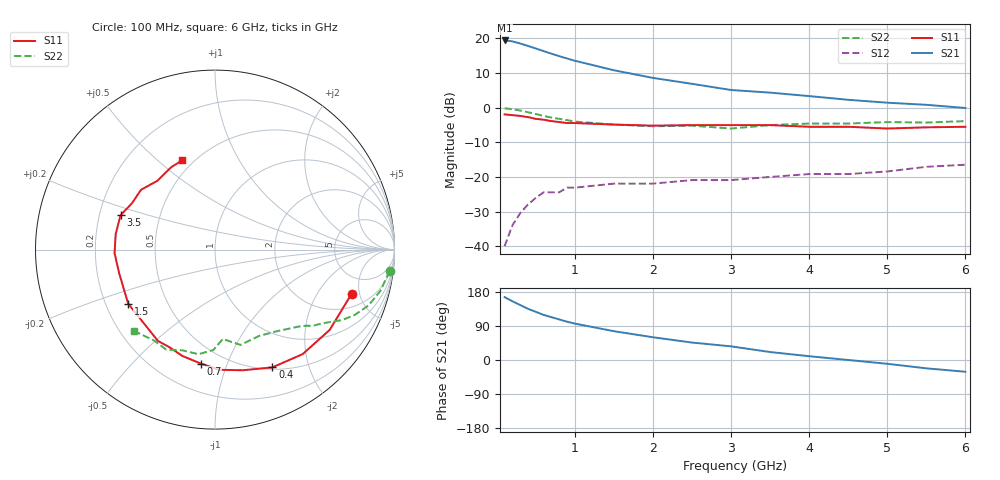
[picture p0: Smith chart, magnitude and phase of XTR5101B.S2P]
! HXTR-5101  (2N6701) Common Emitter
! Vce=15V  Ic=15mA
# ghz s ma r 50
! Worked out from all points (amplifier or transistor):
!   20 points, 100 MHz to 6 GHz, reference 50 ohm
!   highest |S21| = 19.4 dB at 100 MHz (marker M1)
!   |S21| within 3 dB of that: start of sweep to 589.7 MHz
!   unconditionally stable (mu >= 1): 1.896 GHz to end of sweep
!   at 400 MHz: K = 0.25, MSG = 22.9 dB, |S12| = -28.0 dB
!   at 1.5 GHz: K = 0.79, MSG = 16.4 dB, |S12| = -21.9 dB
!   at 6 GHz: K = 1.17, MAG = 5.7 dB, |S12| = -16.5 dB
!   S11 on the Smith chart (normalised r, x): 100 MHz: 3.04, -4.18; 400 MHz: 0.52, -1.47; 700 MHz: 0.38, -0.81; 1.5 GHz: 0.29, -0.26; 3.5 GHz: 0.29, +0.16; 6 GHz: 0.44, +0.61
0.1  0.8 -18.0  9.35 166.0  0.01 78.0  0.98 -7.0
0.2  0.78 -35.0  9.07 155.0  0.02 69.0  0.95 -14.0
0.3  0.76 -50.0  8.44 145.0  0.03 61.0  0.91 -20.0
0.4  0.73 -64.0  7.79 135.0  0.04 55.0  0.86 -25.0
0.5  0.69 -77.0  7.16 127.0  0.05 49.0  0.81 -29.0
0.6  0.67 -88.0  6.56 119.0  0.06 44.0  0.76 -32.0
0.7  0.64 -97.0  6.02 113.0  0.06 40.0  0.72 -35.0
0.8  0.62 -107.0  5.54 107.0  0.06 37.0  0.69 -38.0
0.9  0.6 -115.0  5.13 101.0  0.07 34.0  0.66 -40.0
1  0.6 -122.0  4.76 96.0  0.07 32.0  0.63 -43.0
1.5  0.57 -148.0  3.47 76.0  0.08 24.0  0.57 -53.0
2  0.55 -166.0  2.69 60.0  0.08 21.0  0.54 -63.0
2.5  0.56 -178.0  2.21 46.0  0.09 19.0  0.55 -75.0
3  0.56 171.0  1.8 36.0  0.09 21.0  0.5 -85.0
3.5  0.56 160.0  1.65 21.0  0.1 18.0  0.56 -91.0
4  0.53 151.0  1.47 10.0  0.11 18.0  0.59 -99.0
4.5  0.53 141.0  1.3 0.0  0.11 17.0  0.59 -108.0
5  0.5 130.0  1.18 -10.0  0.12 15.0  0.62 -116.0
5.5  0.52 118.0  1.1 -22.0  0.14 13.0  0.61 -124.0
6  0.53 110.0  0.99 -31.0  0.15 11.0  0.64 -135.0
